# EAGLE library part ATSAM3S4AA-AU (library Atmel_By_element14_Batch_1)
Flash MCU
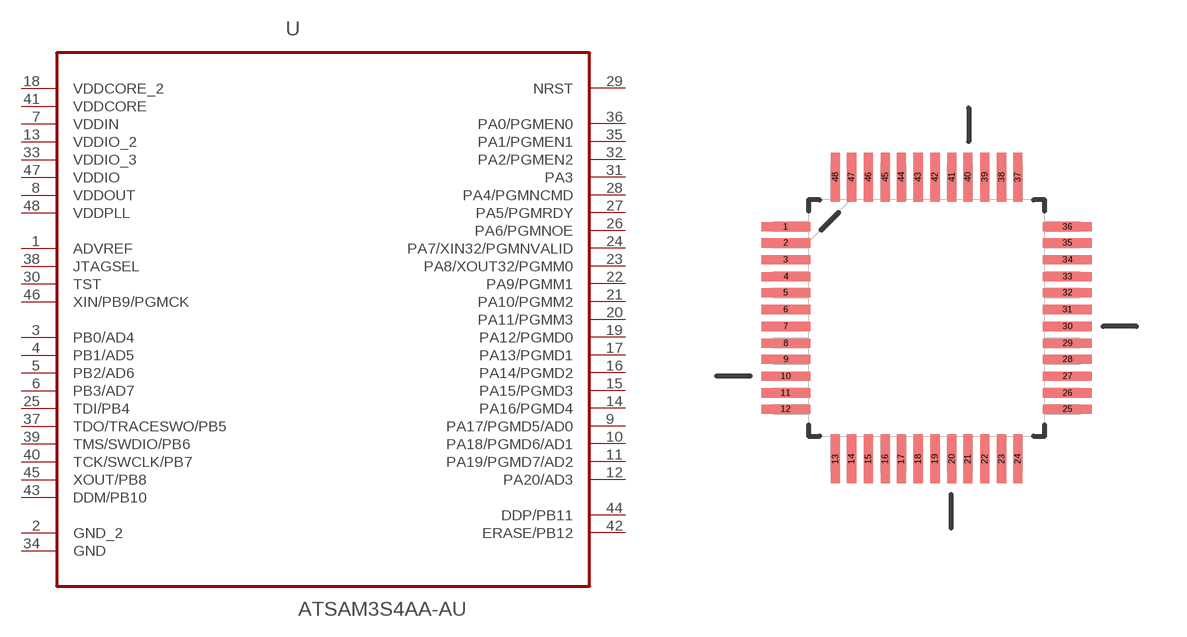
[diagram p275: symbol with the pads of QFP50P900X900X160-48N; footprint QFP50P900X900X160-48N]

Designator prefix U

## ATSAM3S4AA-AU (DESCRIPTION: Flash MCU; MPN: ATSAM3S4AA-AU; OC_FARNELL: 1841655; OC_NEWARK: 12T1313; PACKAGE: QFP-48; SUPPLIER: Atmel)  [QFP50P900X900X160-48N]
1  ADVREF  in
2  GND_2  pas
3  PB0/AD4
4  PB1/AD5
5  PB2/AD6
6  PB3/AD7
7  VDDIN  pwr
8  VDDOUT  pwr
9  PA17/PGMD5/AD0
10  PA18/PGMD6/AD1
11  PA19/PGMD7/AD2
12  PA20/AD3
13  VDDIO_2  pwr
14  PA16/PGMD4
15  PA15/PGMD3
16  PA14/PGMD2
17  PA13/PGMD1
18  VDDCORE_2  pwr
19  PA12/PGMD0
20  PA11/PGMM3
21  PA10/PGMM2
22  PA9/PGMM1
23  PA8/XOUT32/PGMM0
24  PA7/XIN32/PGMNVALID
25  TDI/PB4
26  PA6/PGMNOE
27  PA5/PGMRDY
28  PA4/PGMNCMD
29  NRST
30  TST  in
31  PA3
32  PA2/PGMEN2
33  VDDIO_3  pwr
34  GND  pas
35  PA1/PGMEN1
36  PA0/PGMEN0
37  TDO/TRACESWO/PB5
38  JTAGSEL  in
39  TMS/SWDIO/PB6
40  TCK/SWCLK/PB7
41  VDDCORE  pwr
42  ERASE/PB12
43  DDM/PB10
44  DDP/PB11
45  XOUT/PB8  out
46  XIN/PB9/PGMCK  in
47  VDDIO  pwr
48  VDDPLL  pwr

## Footprint QFP50P900X900X160-48N (pad centres in mm)
smd 1.473 x 0.279: 1 -4.242,2.743; 2 -4.242,2.261; 3 -4.242,1.753; 4 -4.242,1.245; 5 -4.242,0.762; 6 -4.242,0.254; 7 -4.242,-0.254; 8 -4.242,-0.762; 9 -4.242,-1.245; 10 -4.242,-1.753; 11 -4.242,-2.261; 12 -4.242,-2.743; 25 4.242,-2.743; 26 4.242,-2.261; 27 4.242,-1.753; 28 4.242,-1.245; 29 4.242,-0.762; 30 4.242,-0.254; 31 4.242,0.254; 32 4.242,0.762; 33 4.242,1.245; 34 4.242,1.753; 35 4.242,2.261; 36 4.242,2.743
smd 0.279 x 1.473: 13 -2.743,-4.242; 14 -2.261,-4.242; 15 -1.753,-4.242; 16 -1.245,-4.242; 17 -0.762,-4.242; 18 -0.254,-4.242; 19 0.254,-4.242; 20 0.762,-4.242; 21 1.245,-4.242; 22 1.753,-4.242; 23 2.261,-4.242; 24 2.743,-4.242; 37 2.743,4.242; 38 2.261,4.242; 39 1.753,4.242; 40 1.245,4.242; 41 0.762,4.242; 42 0.254,4.242; 43 -0.254,4.242; 44 -0.762,4.242; 45 -1.245,4.242; 46 -1.753,4.242; 47 -2.261,4.242; 48 -2.743,4.242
